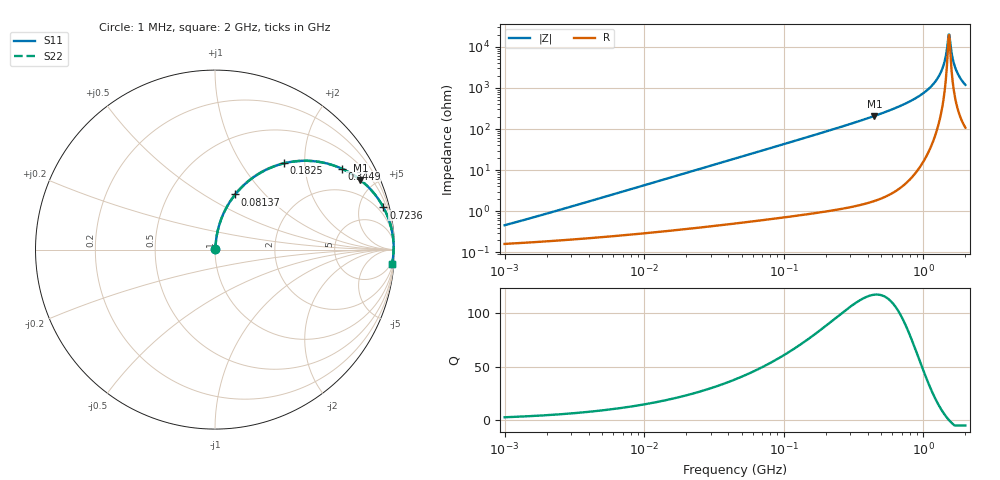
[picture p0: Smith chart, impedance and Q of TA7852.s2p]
# MHz S MA R 50
!Freq  MagS11  AngS11  MagS21  AngS21  MagS12  AngS12  MagS22  AngS22
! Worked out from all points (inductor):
!   801 points, 1 MHz to 2 GHz, reference 50 ohm
!   read as one part in series: L = 68 nH near 1.164 MHz
!   highest Q = 118 at 445.7 MHz (marker M1), where L = 74.3 nH
!   self-resonance near 1.518 GHz
!   S11 on the Smith chart (normalised r, x): 1 MHz: 1.00, +0.01; 81.37 MHz: 1.01, +0.70; 182.5 MHz: 1.02, +1.58; 344.9 MHz: 1.03, +3.11; 723.6 MHz: 1.09, +7.98; 2 GHz: 3, -24
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1  0.004555 69.2  0.9984 -0.2  0.9984 -0.2  0.004555 69.2
3.572091  0.01538 81.2  0.9978 -0.9  0.9978 -0.9  0.01538 81.2
12.63918  0.05385 83.6  0.9954 -3.1  0.9954 -3.1  0.05385 83.6
45.14829  0.1887 77.6  0.9771 -10.9  0.9771 -10.9  0.1887 77.6
81.37127  0.3274 69.8  0.9389 -19.1  0.9389 -19.1  0.3274 69.8
159.7488  0.5647 54.9  0.8182 -34.4  0.8182 -34.4  0.5647 54.9
182.4759  0.6168 51.2  0.7798 -38.1  0.7798 -38.1  0.6168 51.2
344.879  0.8374 32.6  0.5392 -56.9  0.5392 -56.9  0.8374 32.6
445.7348  0.8984 25.6  0.4315 -64.0  0.4315 -64.0  0.8984 25.6
565.2411  0.9391 19.6  0.3355 -69.9  0.3355 -69.9  0.9391 19.6
723.6311  0.9675 14.0  0.2426 -75.3  0.2426 -75.3  0.9675 14.0
990.1129  0.988 7.8  0.1353 -81.0  0.1353 -81.0  0.988 7.8
1220.29  0.9942 3.9  0.06886 -83.2  0.06886 -83.2  0.9942 3.9
1367.661  0.9954 1.9  0.03381 -81.2  0.03381 -81.2  0.9954 1.9
1420.639  0.9955 1.3  0.02234 -77.7  0.02234 -77.7  0.9955 1.3
1489.756  0.9954 0.4  0.008716 -57.8  0.008716 -57.8  0.9954 0.4
1518.335  0.9953 0.1  0.004992 -18.8  0.004992 -18.8  0.9953 0.1
1562.236  0.995 -0.4  0.008632 54.7  0.008632 54.7  0.995 -0.4
1638.242  0.9944 -1.2  0.02221 74.8  0.02221 74.8  0.9944 -1.2
1717.946  0.9936 -2.1  0.03653 78.8  0.03653 78.8  0.9936 -2.1
1853.616  0.9916 -3.4  0.05973 80.2  0.05973 80.2  0.9916 -3.4
2000  0.989 -4.8  0.0832 80.0  0.0832 80.0  0.989 -4.8
